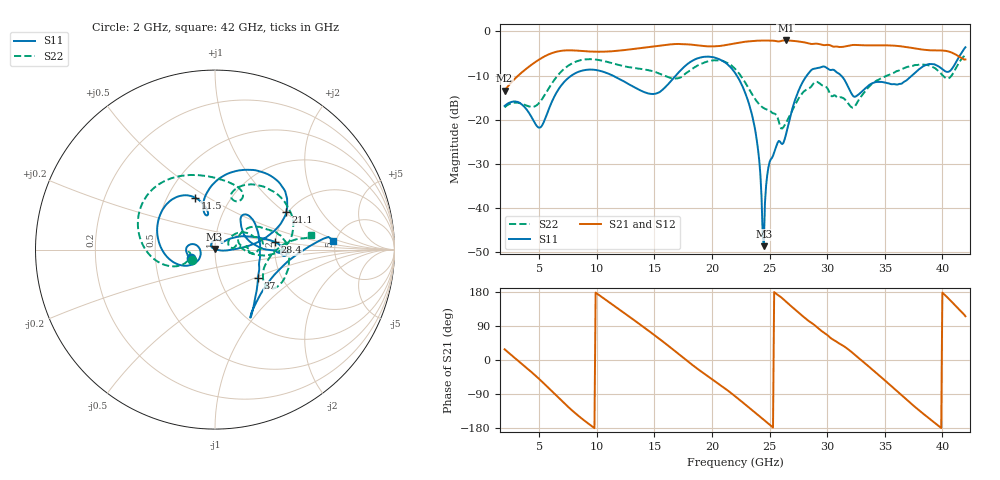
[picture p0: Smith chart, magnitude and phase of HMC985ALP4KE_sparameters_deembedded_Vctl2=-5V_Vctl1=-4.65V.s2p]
!s2p File: Measurements: S11, S21, S12, S22
# GHz S dB R 50.0
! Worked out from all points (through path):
!   401 points, 2 GHz to 42 GHz, reference 50 ohm
!   highest |S21| = -2.06 dB at 26.4 GHz (marker M1); lowest = -13.4 dB at 2 GHz (marker M2)
!   lowest |S11| = -48.6 dB at 24.5 GHz (marker M3), VSWR 1.01, Z = 49.8 + j0.295 ohm
!   |S11| at or under -10 dB: start of sweep to 7.807 GHz; 22.15 GHz to 28.23 GHz (6.082 GHz wide, 24.1 % of centre); 31.21 GHz to 37.36 GHz (6.153 GHz wide, 17.9 % of centre)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
!   |S22| runs from -22.0 to -5.3 dB; largest |S21 - S12| = 0.00086
!   S11 on the Smith chart (normalised r, x): 2 GHz: 0.76, -0.07; 11.5 GHz: 0.68, +0.44; 21.1 GHz: 1.96, +1.02; 28.4 GHz: 2.00, +0.19; 37 GHz: 1.52, -0.52; 42 GHz: 4.73, +0.85
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2  -16.87 -161.7  -13.43 28.3  -13.44 28.3  -17.18 -155.6
5  -21.79 -172.4  -6.37 -50.1  -6.38 -50.1  -16.18 -159.7
6.3  -14.84 -150.3  -4.76 -88.3  -4.76 -88.3  -11.03 -161.5
8.7  -8.91 150.4  -4.44 -154.5  -4.44 -154.5  -6.47 151.3
11.5  -10.15 111.1  -4.47 143.2  -4.47 143.2  -7.32 105.2
13.6  -13.11 101.2  -3.85 97.2  -3.86 97.3  -8.42 75.8
15.4  -13.81 105.8  -3.26 56.6  -3.26 56.6  -9.51 62.2
17.9  -7.34 80.3  -2.95 -3.4  -2.95 -3.4  -9.19 72.2
21.1  -6.97 27.6  -3.14 -74.3  -3.14 -74.2  -6.87 16.2
22  -9.37 17.1  -2.71 -95.4  -2.71 -95.4  -8.46 0.8
23.6  -20.30 -0.0  -2.18 -135.1  -2.18 -135.1  -14.72 -4.1
24.5  -48.58 127.2  -2.08 -157.8  -2.08 -157.8  -17.37 8.3
25  -29.59 133.3  -2.11 -170.5  -2.11 -170.5  -17.93 10.9
26.4  -23.58 42.3  -2.06 154.8  -2.06 154.8  -20.83 33.2
28.4  -9.43 7.2  -2.73 102.9  -2.73 102.9  -12.89 18.6
28.7  -8.61 2.2  -2.86 96.6  -2.86 96.7  -12.19 16.7
30.7  -8.96 -2.9  -3.45 50.9  -3.45 50.9  -14.51 2.6
32.5  -14.70 32.3  -3.09 11.1  -3.09 11.1  -16.58 28.1
35.4  -11.81 19.3  -3.18 -64.4  -3.18 -64.4  -9.81 19.6
37  -10.84 -33.3  -3.60 -107.5  -3.60 -107.5  -8.02 5.3
39.8  -8.15 -57.0  -4.32 -176.9  -4.31 -176.9  -9.32 -35.1
42  -3.60 4.4  -6.37 115.4  -6.37 115.5  -5.34 8.9
